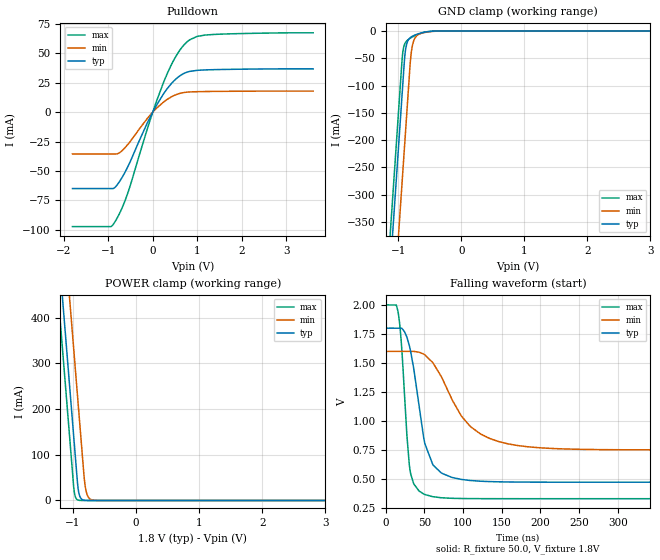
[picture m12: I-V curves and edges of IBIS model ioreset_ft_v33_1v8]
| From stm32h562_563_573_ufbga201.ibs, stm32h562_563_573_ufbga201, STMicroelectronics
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[Model]   ioreset_ft_v33_1v8
Model_type I/O_open_drain
Polarity   Inverting
Enable   Active-Low
| CAP_THRESHOLD on pad IOFT is "UDTCAPC" :
| Rising=20.0% of vddiom   Falling=80.0% of vddiom
| C_comp min and max val. don't necessarily correlate with the min and max pvt
| but are the smallest and greatest pad capacitance found.
| var   typ   min   max
C_comp   3.16940pF  3.14035pF  3.18100pF
|C_comp_pulldown   3.16940pF  3.14035pF  3.18100pF
Vinl = 800.0mV
Vinh = 1.0V
Vmeas = 900.0mV   | Reference voltage for timing measurements
Cref  = 50.0pF   | Timing specification test load capacitance value
Rref  = 1.0MOhm   | Timing specification test load resistance value
Vref  = 990.0mV   | Timing specification test load voltage
[Model Spec]
| TIME_THRESHOLD on pin ZIV33M is "CMOS" :
| Rising=40.0% of vddiom   Falling=60.0% of vddiom
Vinl 699.80000mV 627.80000mV 779.80000mV
Vinh 1.05220V 928.20000mV 1.15620V
| variable   typ   min   max
[Temperature Range] 25.0 125.0 -40.0
| variable   typ   min   max
[Voltage Range] 1.8V 1.6V 2.0V
| variable   typ   min   max
[POWER Clamp Reference] 1.8V 1.6V 2.0V
| variable   typ   min   max
[GND Clamp Reference] 0V 0V 0V
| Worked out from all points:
|   slope of the pulldown table from 0 to 0.27 V, typ, clamps not added: 15.8 ohm
|   GND clamp passes 1 mA (typ) near -0.52 V on its own axis
|   POWER clamp passes 1 mA (typ) near -0.84 V on its own axis
|   falling waveform, R_fixture 50.0, V_fixture 1.8V: 20-80 % time 20.4ns typ, 48.4ns min, 9.75ns max; typ from 1.8 V to 0.474 V
[POWER Clamp]
-1.8V     1.518A     1.709A     1.407A
-1.24V    565.8mA    757.2mA    454.5mA
-1.18V    463.8mA    655.2mA    352.5mA
-1.11V    344.8mA    536.2mA    233.5mA
-1.05V    242.8mA    434.2mA    131.5mA
-980mV    123.8mA    315.2mA    17.95mA
-930mV    38.81mA    230.2mA    1.49mA
-890mV    8.18mA     162.2mA    203.5uA
-810mV    363.5uA    33.6mA     3.797uA
-770mV    76.62uA    10.47mA    518.7nA
-710mV    7.416uA    1.822mA    26.23nA
3.6V      0A         0A         0A
[GND Clamp]
-1.8V     -1.579A    -1.74A     -1.515A
-1.24V    -627.3mA   -788.3mA   -562.7mA
-1.05V    -304.3mA   -465.3mA   -239.7mA
-940mV    -117.3mA   -278.3mA   -52.69mA
-930mV    -100.3mA   -261.3mA   -40.52mA
-900mV    -50.11mA   -210.3mA   -24.22mA
-880mV    -30.95mA   -176.3mA   -20.02mA
-810mV    -12.18mA   -57.96mA   -13.22mA
-780mV    -9.803mA   -29.1mA    -11.18mA
-690mV    -5.404mA   -7.14mA    -6.176mA
-420mV    -168.9uA   -443.8uA   -80.87uA
3.6V      312.6pA    43.66nA    94.46pA
| variable   typ   min   max
[Pullup Reference] 1.8V 1.6V 2.0V
| variable   typ   min   max
[Pulldown Reference] 0V 0V 0V
[Pulldown]
-1.8V     -65.01mA   -35.56mA   -97.42mA
-940mV    -65.01mA   -35.56mA   -97.42mA
-850mV    -64.17mA   -35.56mA   -93.5mA
-730mV    -58.19mA   -34.15mA   -85.08mA
-570mV    -47.32mA   -28.01mA   -70.04mA
-120mV    -9.088mA   -5.279mA   -14.07mA
250mV     16.04mA    8.832mA    26.05mA
520mV     28.19mA    14.82mA    47.53mA
780mV     34.17mA    17.07mA    60.14mA
1V        35.61mA    17.44mA    64.53mA
1.37V     36.18mA    17.65mA    66.15mA
3.6V      36.85mA    17.91mA    67.54mA
[Ramp]
dV/dt_r 793.63753mV/454.81899ps 509.89008mV/978.78162ps 1.00535V/290.26081ps
dV/dt_f 795.78722mV/18.98959ns 508.98182mV/47.36521ns 1.00093V/9.59494ns
R_load = 50.0
| Removed startup time: 0s 0s 0s  .
| Removed end time: 99.99us.
[Falling Waveform]
R_fixture   = 50.0
V_fixture   = 1.8V
V_fixture_min = 1.6V
V_fixture_max = 2.0V
0s        1.8V       1.6V       2V
16.35ns   1.8V       1.6V       1.927V
20.7ns    1.799V     1.6V       1.63V
27.55ns   1.721V     1.6V       868mV
35.85ns   1.469V     1.6V       467.7mV
50.65ns   805.5mV    1.571V     367.7mV
71.5ns    555.9mV    1.388V     340.1mV
108ns     489.4mV    963.7mV    332.6mV
158.8ns   475.7mV    802.9mV    331.7mV
598.7ns   473.7mV    751.7mV    331.7mV
